(* Logix 5000 AddOnInstructionDefinition export Banner_Q90R2KU_Param_v4; software revision 33.00; part 2 of 3 *)
(* tags used below, declared in another part *)
   Q90RKU : Banner_Q90R2KU_v4;
   Port_Data : Banner_IOL_Port_v4;
   Port : DINT;
   Local_Control : DINT;
   Command_Being_Processed : BOOL;
   Update_Archive : BOOL;
   Index_Write_Inprocess : DINT;
   Index_Write_Control : DINT;
   Inprocess_Index : DINT;
(* Banner_Q90R2KU_Param_v4, continued *)

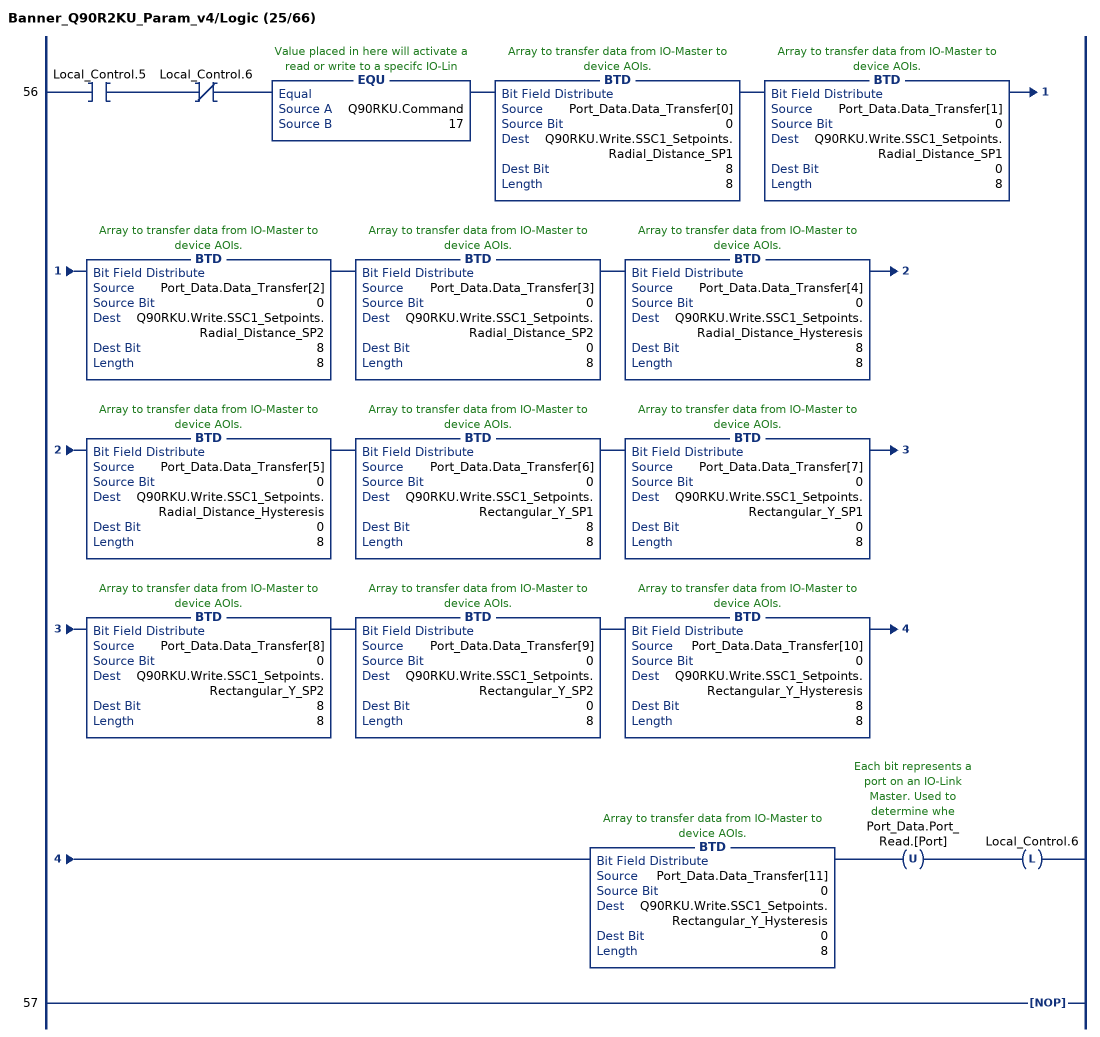
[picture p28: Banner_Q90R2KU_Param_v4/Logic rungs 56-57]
   56: XIC(Local_Control.5)XIO(Local_Control.6)EQU(Q90RKU.Command,17)BTD(Port_Data.Data_Transfer[0],0,Q90RKU.Write.SSC1_Setpoints.Radial_Distance_SP1,8,8)BTD(Port_Data.Data_Transfer[1],0,Q90RKU.Write.SSC1_Setpoints.Radial_Distance_SP1,0,8)BTD(Port_Data.Data_Transfer[2],0,Q90RKU.Write.SSC1_Setpoints.Radial_Distance_SP2,8,8)BTD(Port_Data.Data_Transfer[3],0,Q90RKU.Write.SSC1_Setpoints.Radial_Distance_SP2,0,8)BTD(Port_Data.Data_Transfer[4],0,Q90RKU.Write.SSC1_Setpoints.Radial_Distance_Hysteresis,8,8)BTD(Port_Data.Data_Transfer[5],0,Q90RKU.Write.SSC1_Setpoints.Radial_Distance_Hysteresis,0,8)BTD(Port_Data.Data_Transfer[6],0,Q90RKU.Write.SSC1_Setpoints.Rectangular_Y_SP1,8,8)BTD(Port_Data.Data_Transfer[7],0,Q90RKU.Write.SSC1_Setpoints.Rectangular_Y_SP1,0,8)BTD(Port_Data.Data_Transfer[8],0,Q90RKU.Write.SSC1_Setpoints.Rectangular_Y_SP2,8,8)BTD(Port_Data.Data_Transfer[9],0,Q90RKU.Write.SSC1_Setpoints.Rectangular_Y_SP2,0,8)BTD(Port_Data.Data_Transfer[10],0,Q90RKU.Write.SSC1_Setpoints.Rectangular_Y_Hysteresis,8,8)BTD(Port_Data.Data_Transfer[11],0,Q90RKU.Write.SSC1_Setpoints.Rectangular_Y_Hysteresis,0,8)OTU(Port_Data.Port_Read.[Port])OTL(Local_Control.6);
   57: NOP();
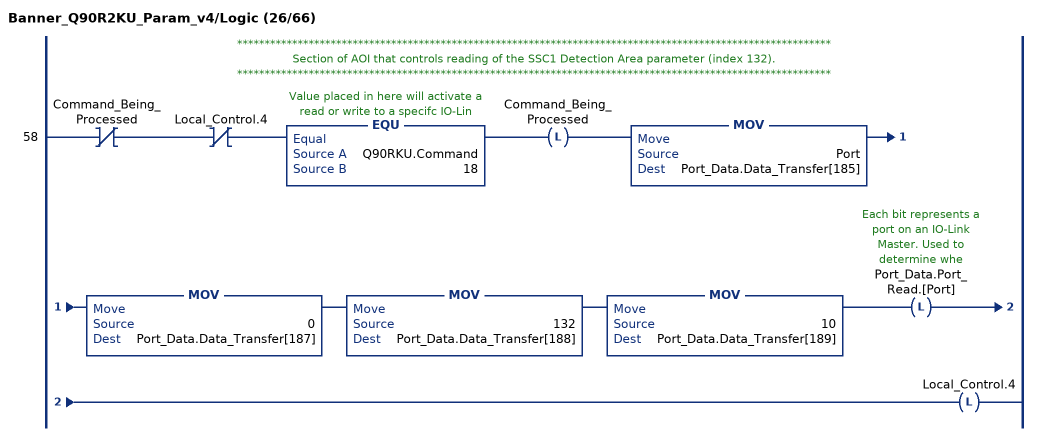
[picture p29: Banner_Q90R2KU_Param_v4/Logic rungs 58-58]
   // ************************************************************************************************************
   // Section of AOI that controls reading of the SSC1 Detection Area parameter (index 132).
   // ************************************************************************************************************
   58: XIO(Command_Being_Processed)XIO(Local_Control.4)EQU(Q90RKU.Command,18)OTL(Command_Being_Processed)MOV(Port,Port_Data.Data_Transfer[185])MOV(0,Port_Data.Data_Transfer[187])MOV(132,Port_Data.Data_Transfer[188])MOV(10,Port_Data.Data_Transfer[189])OTL(Port_Data.Port_Read.[Port])OTL(Local_Control.4);
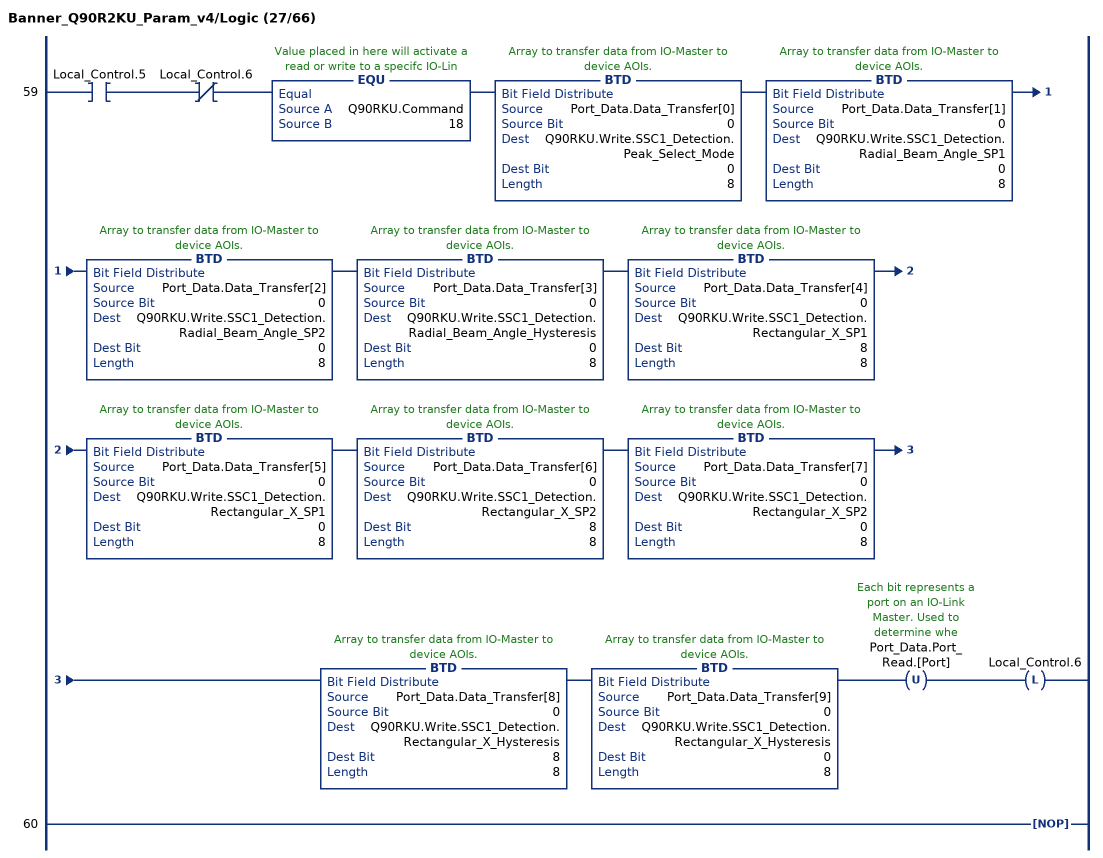
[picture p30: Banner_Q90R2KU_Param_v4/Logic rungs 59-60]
   59: XIC(Local_Control.5)XIO(Local_Control.6)EQU(Q90RKU.Command,18)BTD(Port_Data.Data_Transfer[0],0,Q90RKU.Write.SSC1_Detection.Peak_Select_Mode,0,8)BTD(Port_Data.Data_Transfer[1],0,Q90RKU.Write.SSC1_Detection.Radial_Beam_Angle_SP1,0,8)BTD(Port_Data.Data_Transfer[2],0,Q90RKU.Write.SSC1_Detection.Radial_Beam_Angle_SP2,0,8)BTD(Port_Data.Data_Transfer[3],0,Q90RKU.Write.SSC1_Detection.Radial_Beam_Angle_Hysteresis,0,8)BTD(Port_Data.Data_Transfer[4],0,Q90RKU.Write.SSC1_Detection.Rectangular_X_SP1,8,8)BTD(Port_Data.Data_Transfer[5],0,Q90RKU.Write.SSC1_Detection.Rectangular_X_SP1,0,8)BTD(Port_Data.Data_Transfer[6],0,Q90RKU.Write.SSC1_Detection.Rectangular_X_SP2,8,8)BTD(Port_Data.Data_Transfer[7],0,Q90RKU.Write.SSC1_Detection.Rectangular_X_SP2,0,8)BTD(Port_Data.Data_Transfer[8],0,Q90RKU.Write.SSC1_Detection.Rectangular_X_Hysteresis,8,8)BTD(Port_Data.Data_Transfer[9],0,Q90RKU.Write.SSC1_Detection.Rectangular_X_Hysteresis,0,8)OTU(Port_Data.Port_Read.[Port])OTL(Local_Control.6);
   60: NOP();
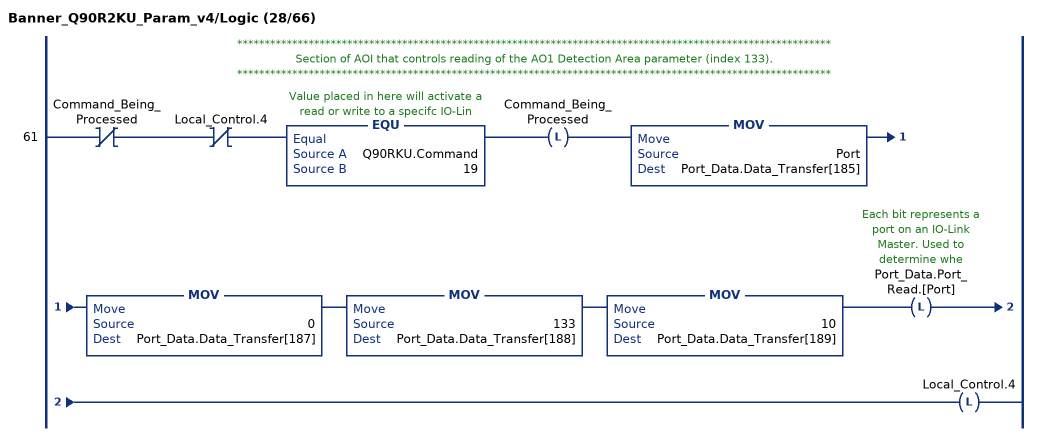
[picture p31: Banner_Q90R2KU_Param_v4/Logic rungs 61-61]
   // ************************************************************************************************************
   // Section of AOI that controls reading of the AO1 Detection Area parameter (index 133).
   // ************************************************************************************************************
   61: XIO(Command_Being_Processed)XIO(Local_Control.4)EQU(Q90RKU.Command,19)OTL(Command_Being_Processed)MOV(Port,Port_Data.Data_Transfer[185])MOV(0,Port_Data.Data_Transfer[187])MOV(133,Port_Data.Data_Transfer[188])MOV(10,Port_Data.Data_Transfer[189])OTL(Port_Data.Port_Read.[Port])OTL(Local_Control.4);
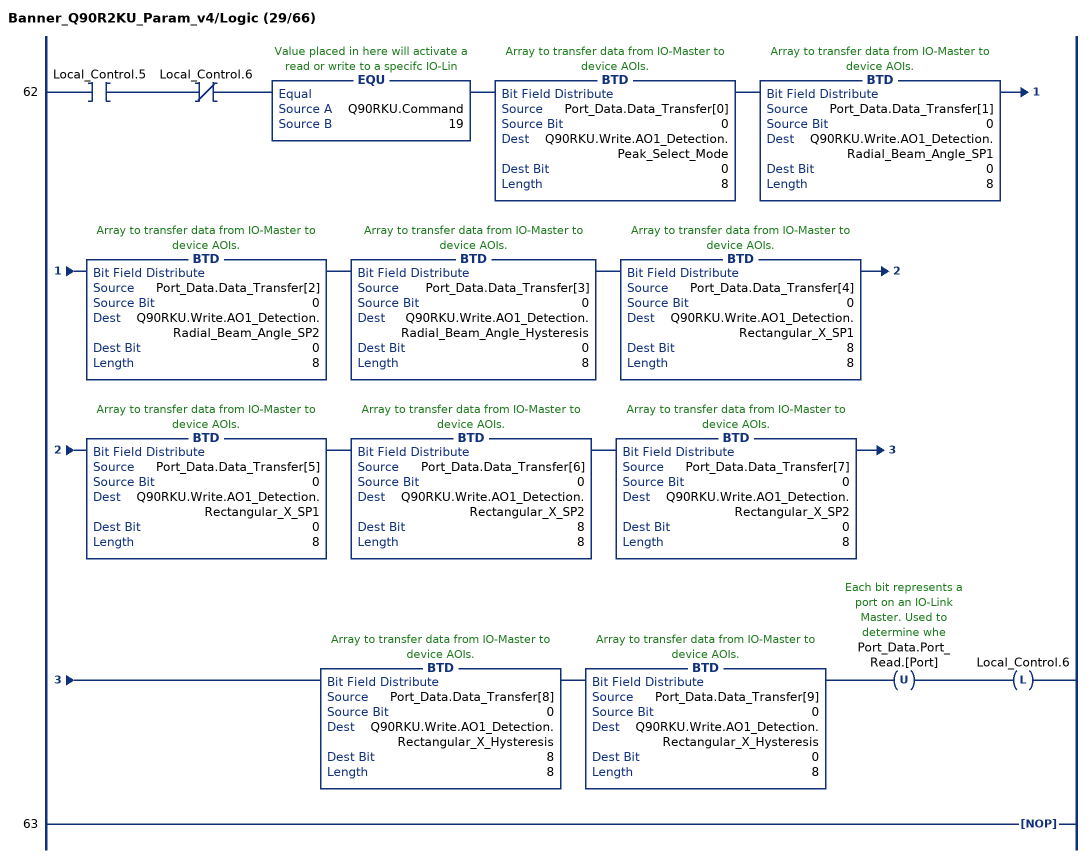
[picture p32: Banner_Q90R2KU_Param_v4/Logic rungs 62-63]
   62: XIC(Local_Control.5)XIO(Local_Control.6)EQU(Q90RKU.Command,19)BTD(Port_Data.Data_Transfer[0],0,Q90RKU.Write.AO1_Detection.Peak_Select_Mode,0,8)BTD(Port_Data.Data_Transfer[1],0,Q90RKU.Write.AO1_Detection.Radial_Beam_Angle_SP1,0,8)BTD(Port_Data.Data_Transfer[2],0,Q90RKU.Write.AO1_Detection.Radial_Beam_Angle_SP2,0,8)BTD(Port_Data.Data_Transfer[3],0,Q90RKU.Write.AO1_Detection.Radial_Beam_Angle_Hysteresis,0,8)BTD(Port_Data.Data_Transfer[4],0,Q90RKU.Write.AO1_Detection.Rectangular_X_SP1,8,8)BTD(Port_Data.Data_Transfer[5],0,Q90RKU.Write.AO1_Detection.Rectangular_X_SP1,0,8)BTD(Port_Data.Data_Transfer[6],0,Q90RKU.Write.AO1_Detection.Rectangular_X_SP2,8,8)BTD(Port_Data.Data_Transfer[7],0,Q90RKU.Write.AO1_Detection.Rectangular_X_SP2,0,8)BTD(Port_Data.Data_Transfer[8],0,Q90RKU.Write.AO1_Detection.Rectangular_X_Hysteresis,8,8)BTD(Port_Data.Data_Transfer[9],0,Q90RKU.Write.AO1_Detection.Rectangular_X_Hysteresis,0,8)OTU(Port_Data.Port_Read.[Port])OTL(Local_Control.6);
   63: NOP();
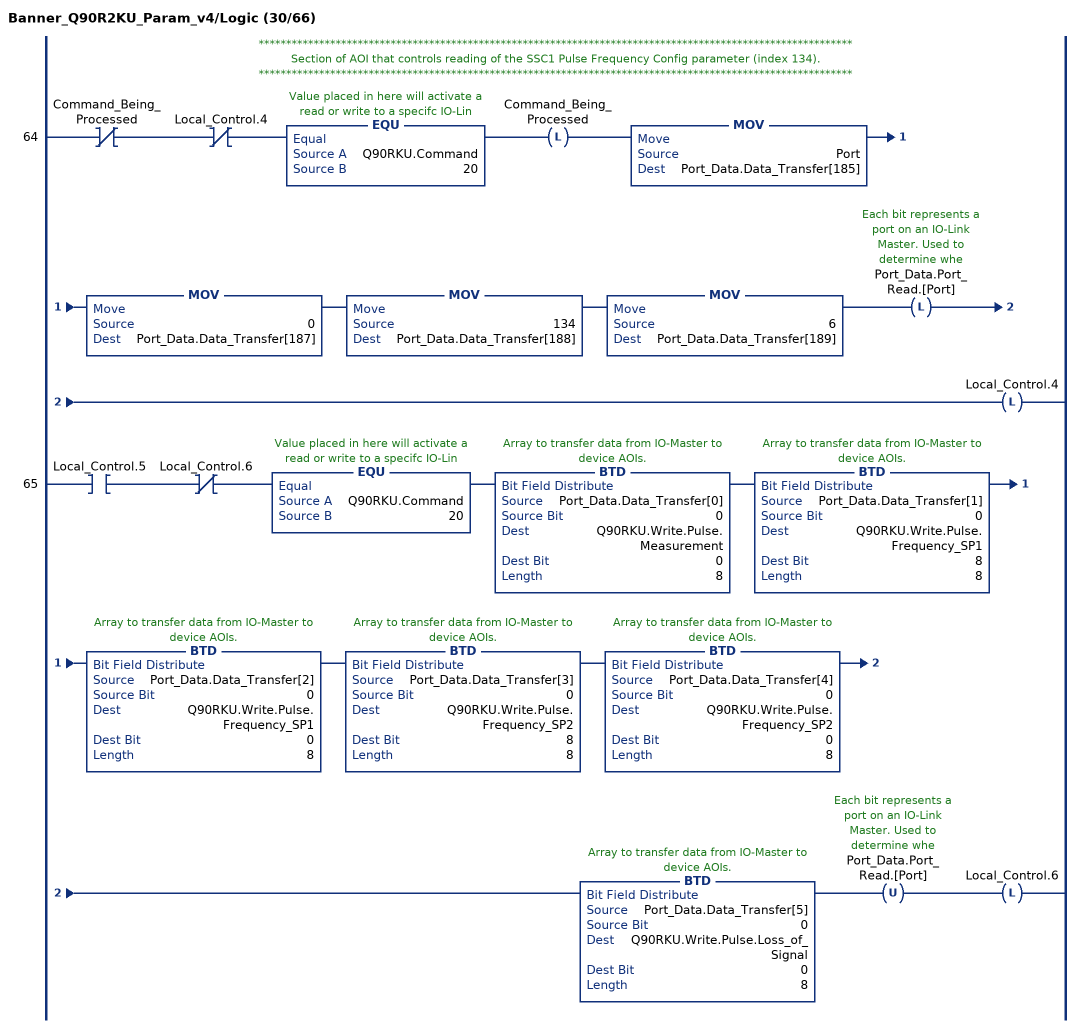
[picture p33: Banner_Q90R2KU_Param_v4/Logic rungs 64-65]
   // ************************************************************************************************************
   // Section of AOI that controls reading of the SSC1 Pulse Frequency Config parameter (index 134).
   // ************************************************************************************************************
   64: XIO(Command_Being_Processed)XIO(Local_Control.4)EQU(Q90RKU.Command,20)OTL(Command_Being_Processed)MOV(Port,Port_Data.Data_Transfer[185])MOV(0,Port_Data.Data_Transfer[187])MOV(134,Port_Data.Data_Transfer[188])MOV(6,Port_Data.Data_Transfer[189])OTL(Port_Data.Port_Read.[Port])OTL(Local_Control.4);
   65: XIC(Local_Control.5)XIO(Local_Control.6)EQU(Q90RKU.Command,20)BTD(Port_Data.Data_Transfer[0],0,Q90RKU.Write.Pulse.Measurement,0,8)BTD(Port_Data.Data_Transfer[1],0,Q90RKU.Write.Pulse.Frequency_SP1,8,8)BTD(Port_Data.Data_Transfer[2],0,Q90RKU.Write.Pulse.Frequency_SP1,0,8)BTD(Port_Data.Data_Transfer[3],0,Q90RKU.Write.Pulse.Frequency_SP2,8,8)BTD(Port_Data.Data_Transfer[4],0,Q90RKU.Write.Pulse.Frequency_SP2,0,8)BTD(Port_Data.Data_Transfer[5],0,Q90RKU.Write.Pulse.Loss_of_Signal,0,8)OTU(Port_Data.Port_Read.[Port])OTL(Local_Control.6);
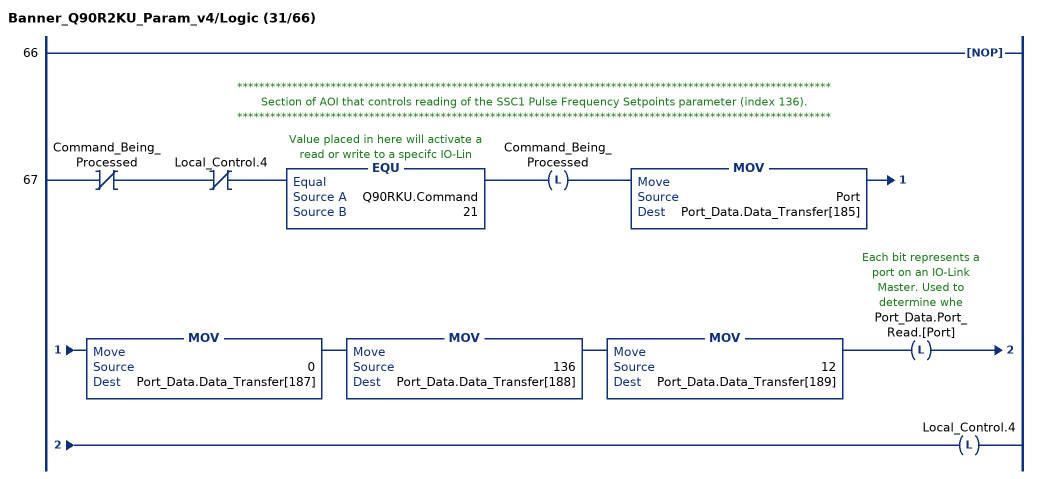
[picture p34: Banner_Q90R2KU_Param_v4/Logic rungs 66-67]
   66: NOP();
   // ************************************************************************************************************
   // Section of AOI that controls reading of the SSC1 Pulse Frequency Setpoints parameter (index 136).
   // ************************************************************************************************************
   67: XIO(Command_Being_Processed)XIO(Local_Control.4)EQU(Q90RKU.Command,21)OTL(Command_Being_Processed)MOV(Port,Port_Data.Data_Transfer[185])MOV(0,Port_Data.Data_Transfer[187])MOV(136,Port_Data.Data_Transfer[188])MOV(12,Port_Data.Data_Transfer[189])OTL(Port_Data.Port_Read.[Port])OTL(Local_Control.4);
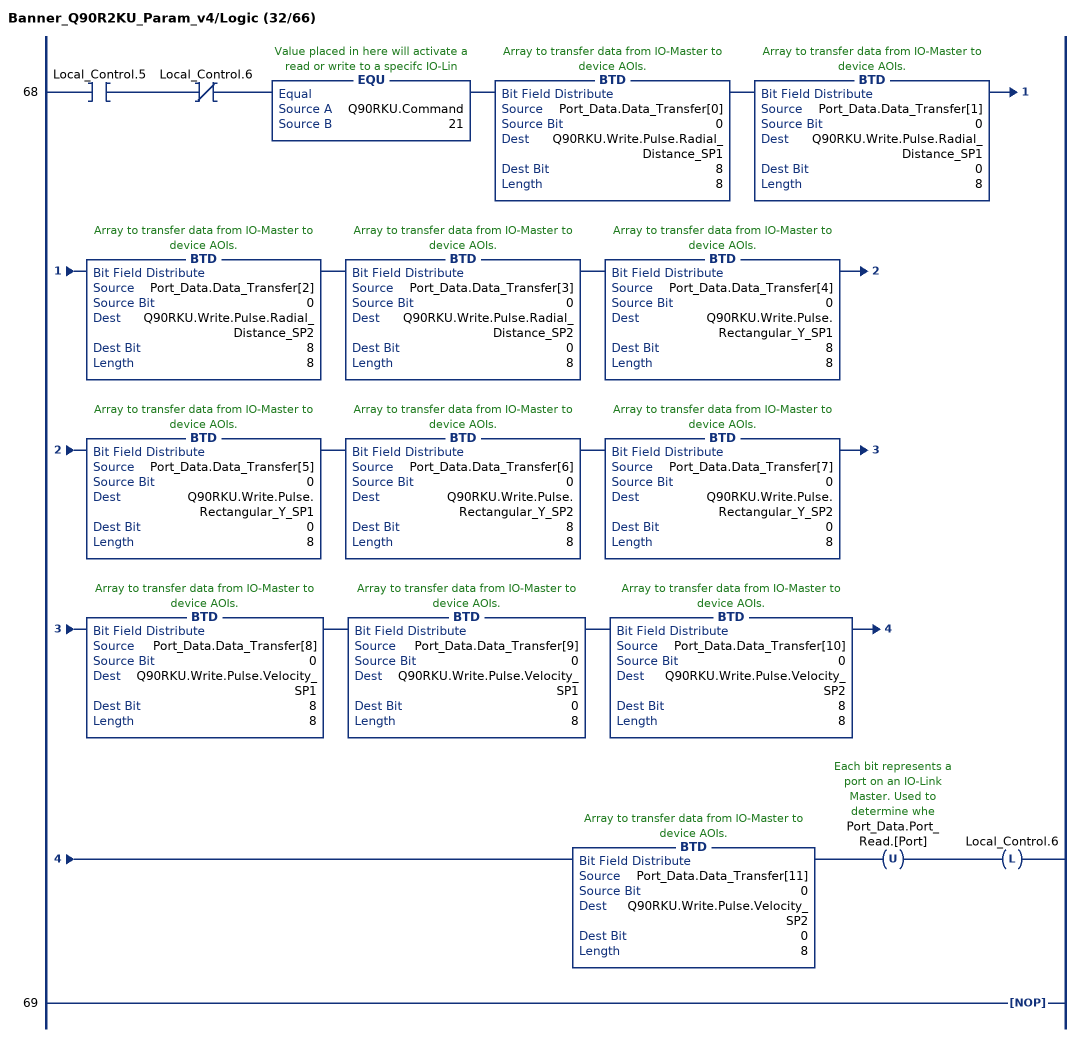
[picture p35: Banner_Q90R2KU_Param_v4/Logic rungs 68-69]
   68: XIC(Local_Control.5)XIO(Local_Control.6)EQU(Q90RKU.Command,21)BTD(Port_Data.Data_Transfer[0],0,Q90RKU.Write.Pulse.Radial_Distance_SP1,8,8)BTD(Port_Data.Data_Transfer[1],0,Q90RKU.Write.Pulse.Radial_Distance_SP1,0,8)BTD(Port_Data.Data_Transfer[2],0,Q90RKU.Write.Pulse.Radial_Distance_SP2,8,8)BTD(Port_Data.Data_Transfer[3],0,Q90RKU.Write.Pulse.Radial_Distance_SP2,0,8)BTD(Port_Data.Data_Transfer[4],0,Q90RKU.Write.Pulse.Rectangular_Y_SP1,8,8)BTD(Port_Data.Data_Transfer[5],0,Q90RKU.Write.Pulse.Rectangular_Y_SP1,0,8)BTD(Port_Data.Data_Transfer[6],0,Q90RKU.Write.Pulse.Rectangular_Y_SP2,8,8)BTD(Port_Data.Data_Transfer[7],0,Q90RKU.Write.Pulse.Rectangular_Y_SP2,0,8)BTD(Port_Data.Data_Transfer[8],0,Q90RKU.Write.Pulse.Velocity_SP1,8,8)BTD(Port_Data.Data_Transfer[9],0,Q90RKU.Write.Pulse.Velocity_SP1,0,8)BTD(Port_Data.Data_Transfer[10],0,Q90RKU.Write.Pulse.Velocity_SP2,8,8)BTD(Port_Data.Data_Transfer[11],0,Q90RKU.Write.Pulse.Velocity_SP2,0,8)OTU(Port_Data.Port_Read.[Port])OTL(Local_Control.6);
   69: NOP();
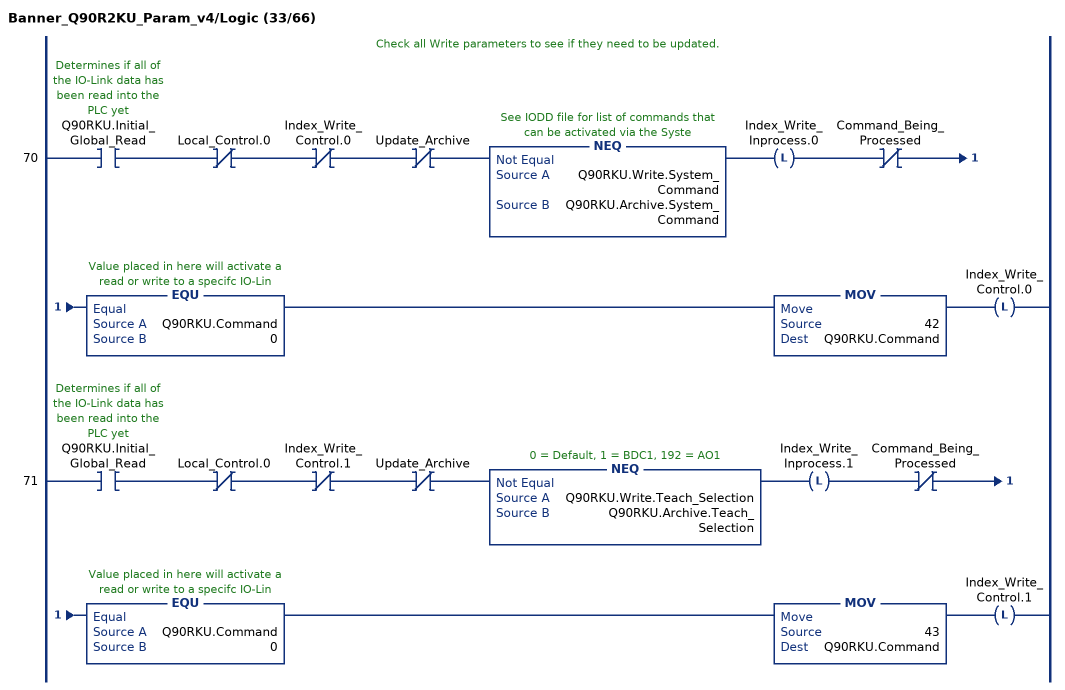
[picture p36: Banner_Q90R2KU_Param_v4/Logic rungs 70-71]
   // Check all Write parameters to see if they need to be updated.
   70: XIC(Q90RKU.Initial_Global_Read)XIO(Local_Control.0)XIO(Index_Write_Control.0)XIO(Update_Archive)NEQ(Q90RKU.Write.System_Command,Q90RKU.Archive.System_Command)OTL(Index_Write_Inprocess.0)XIO(Command_Being_Processed)EQU(Q90RKU.Command,0)MOV(42,Q90RKU.Command)OTL(Index_Write_Control.0);
   71: XIC(Q90RKU.Initial_Global_Read)XIO(Local_Control.0)XIO(Index_Write_Control.1)XIO(Update_Archive)NEQ(Q90RKU.Write.Teach_Selection,Q90RKU.Archive.Teach_Selection)OTL(Index_Write_Inprocess.1)XIO(Command_Being_Processed)EQU(Q90RKU.Command,0)MOV(43,Q90RKU.Command)OTL(Index_Write_Control.1);
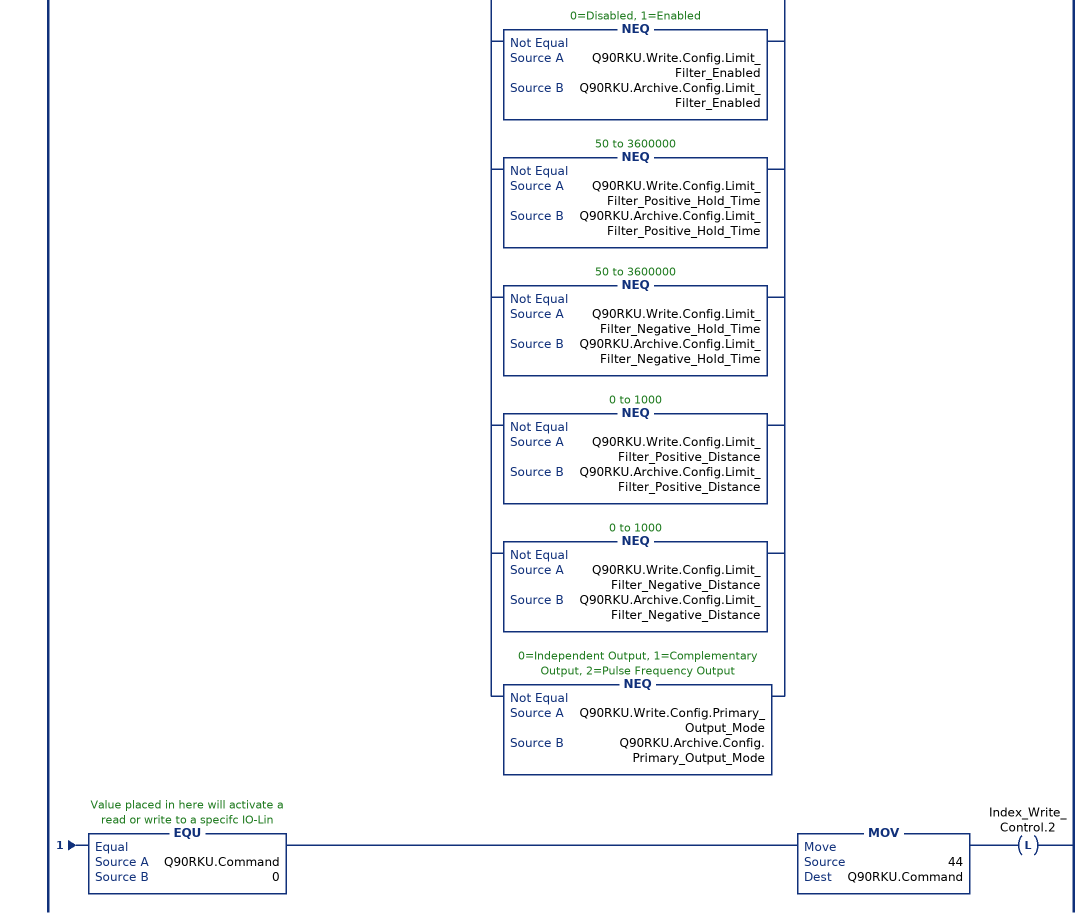
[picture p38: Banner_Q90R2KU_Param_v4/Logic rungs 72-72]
   72: XIC(Q90RKU.Initial_Global_Read)XIO(Local_Control.0)XIO(Index_Write_Control.2)XIO(Update_Archive)[NEQ(Q90RKU.Write.Config.Response_Speed,Q90RKU.Archive.Config.Response_Speed) ,NEQ(Q90RKU.Write.Config.Detection_Sensitivity,Q90RKU.Archive.Config.Detection_Sensitivity) ,NEQ(Q90RKU.Write.Config.LEDs_Disabled,Q90RKU.Archive.Config.LEDs_Disabled) ,NEQ(Q90RKU.Write.Config.Output_Polarity,Q90RKU.Archive.Config.Output_Polarity) ,NEQ(Q90RKU.Write.Config.PD_Measurement,Q90RKU.Archive.Config.PD_Measurement) ,NEQ(Q90RKU.Write.Config.Remote_Input_Mode,Q90RKU.Archive.Config.Remote_Input_Mode) ,NEQ(Q90RKU.Write.Config.Amplitude_Threshold,Q90RKU.Archive.Config.Amplitude_Threshold) ,NEQ(Q90RKU.Write.Config.Limit_Filter_Enabled,Q90RKU.Archive.Config.Limit_Filter_Enabled) ,NEQ(Q90RKU.Write.Config.Limit_Filter_Positive_Hold_Time,Q90RKU.Archive.Config.Limit_Filter_Positive_Hold_Time) ,NEQ(Q90RKU.Write.Config.Limit_Filter_Negative_Hold_Time,Q90RKU.Archive.Config.Limit_Filter_Negative_Hold_Time) ,NEQ(Q90RKU.Write.Config.Limit_Filter_Positive_Distance,Q90RKU.Archive.Config.Limit_Filter_Positive_Distance) ,NEQ(Q90RKU.Write.Config.Limit_Filter_Negative_Distance,Q90RKU.Archive.Config.Limit_Filter_Negative_Distance) ,NEQ(Q90RKU.Write.Config.Primary_Output_Mode,Q90RKU.Archive.Config.Primary_Output_Mode) ]OTL(Index_Write_Inprocess.2)XIO(Command_Being_Processed)EQU(Q90RKU.Command,0)MOV(44,Q90RKU.Command)OTL(Index_Write_Control.2);
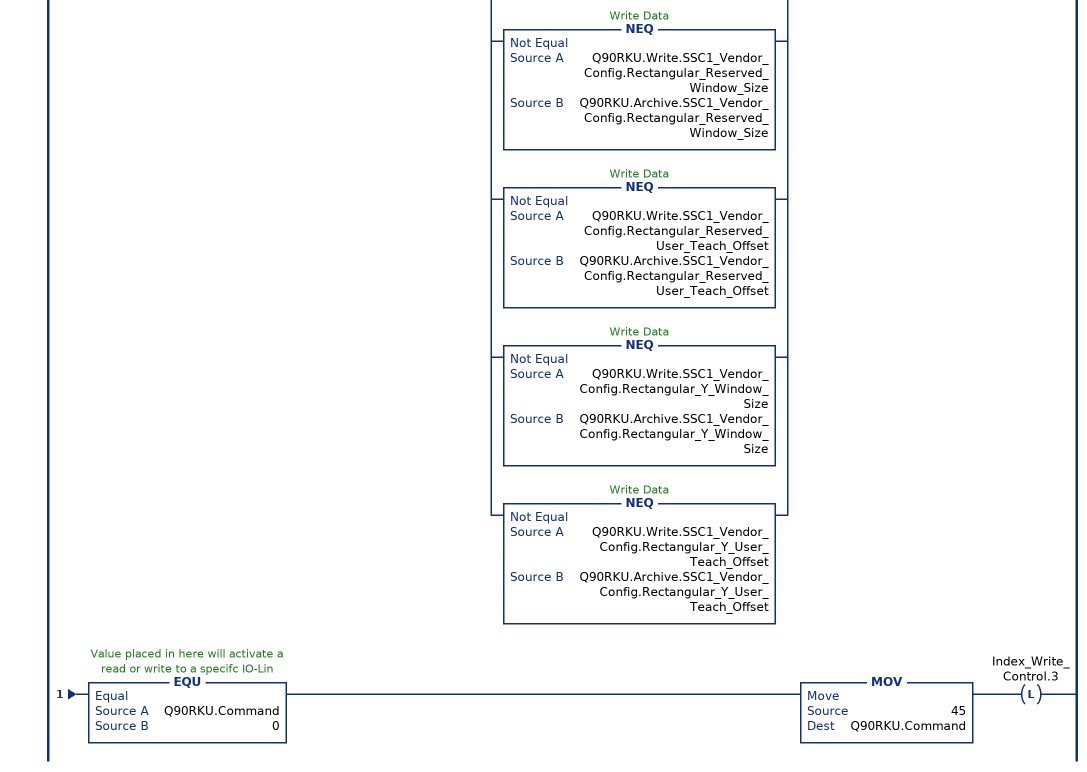
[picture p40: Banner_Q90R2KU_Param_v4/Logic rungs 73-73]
   73: XIC(Q90RKU.Initial_Global_Read)XIO(Local_Control.0)XIO(Index_Write_Control.3)XIO(Update_Archive)[NEQ(Q90RKU.Write.SSC1_Vendor_Config.Delay_On,Q90RKU.Archive.SSC1_Vendor_Config.Delay_On) ,NEQ(Q90RKU.Write.SSC1_Vendor_Config.Delay_Off,Q90RKU.Archive.SSC1_Vendor_Config.Delay_Off) ,NEQ(Q90RKU.Write.SSC1_Vendor_Config.Radial_Distance_Window_Size,Q90RKU.Archive.SSC1_Vendor_Config.Radial_Distance_Window_Size) ,NEQ(Q90RKU.Write.SSC1_Vendor_Config.Radial_Distance_User_Teach_Offset,Q90RKU.Archive.SSC1_Vendor_Config.Radial_Distance_User_Teach_Offset) ,NEQ(Q90RKU.Write.SSC1_Vendor_Config.Radial_Reserved_Window_Size,Q90RKU.Archive.SSC1_Vendor_Config.Radial_Reserved_Window_Size) ,NEQ(Q90RKU.Write.SSC1_Vendor_Config.Radial_Reserved_User_Teach_Offset,Q90RKU.Archive.SSC1_Vendor_Config.Radial_Reserved_User_Teach_Offset) ,NEQ(Q90RKU.Write.SSC1_Vendor_Config.Rectangular_Reserved_Window_Size,Q90RKU.Archive.SSC1_Vendor_Config.Rectangular_Reserved_Window_Size) ,NEQ(Q90RKU.Write.SSC1_Vendor_Config.Rectangular_Reserved_User_Teach_Offset,Q90RKU.Archive.SSC1_Vendor_Config.Rectangular_Reserved_User_Teach_Offset) ,NEQ(Q90RKU.Write.SSC1_Vendor_Config.Rectangular_Y_Window_Size,Q90RKU.Archive.SSC1_Vendor_Config.Rectangular_Y_Window_Size) ,NEQ(Q90RKU.Write.SSC1_Vendor_Config.Rectangular_Y_User_Teach_Offset,Q90RKU.Archive.SSC1_Vendor_Config.Rectangular_Y_User_Teach_Offset) ]OTL(Index_Write_Inprocess.3)XIO(Command_Being_Processed)EQU(Q90RKU.Command,0)MOV(45,Q90RKU.Command)OTL(Index_Write_Control.3);
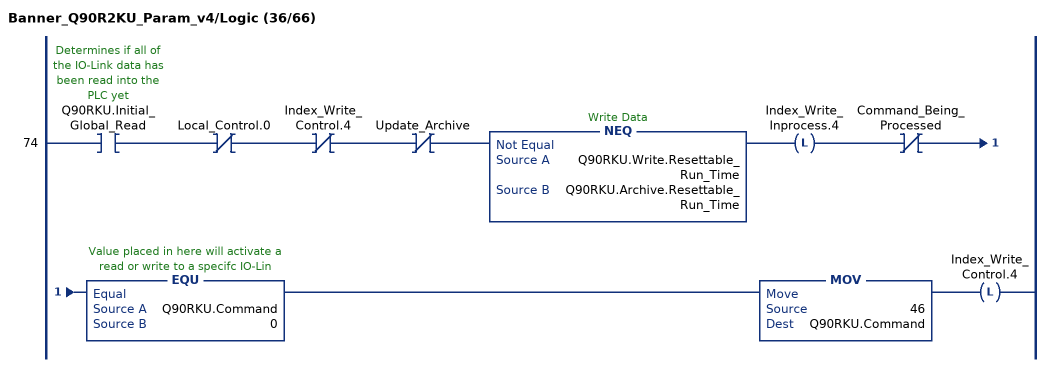
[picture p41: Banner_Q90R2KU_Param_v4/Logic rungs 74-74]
   74: XIC(Q90RKU.Initial_Global_Read)XIO(Local_Control.0)XIO(Index_Write_Control.4)XIO(Update_Archive)NEQ(Q90RKU.Write.Resettable_Run_Time,Q90RKU.Archive.Resettable_Run_Time)OTL(Index_Write_Inprocess.4)XIO(Command_Being_Processed)EQU(Q90RKU.Command,0)MOV(46,Q90RKU.Command)OTL(Index_Write_Control.4);
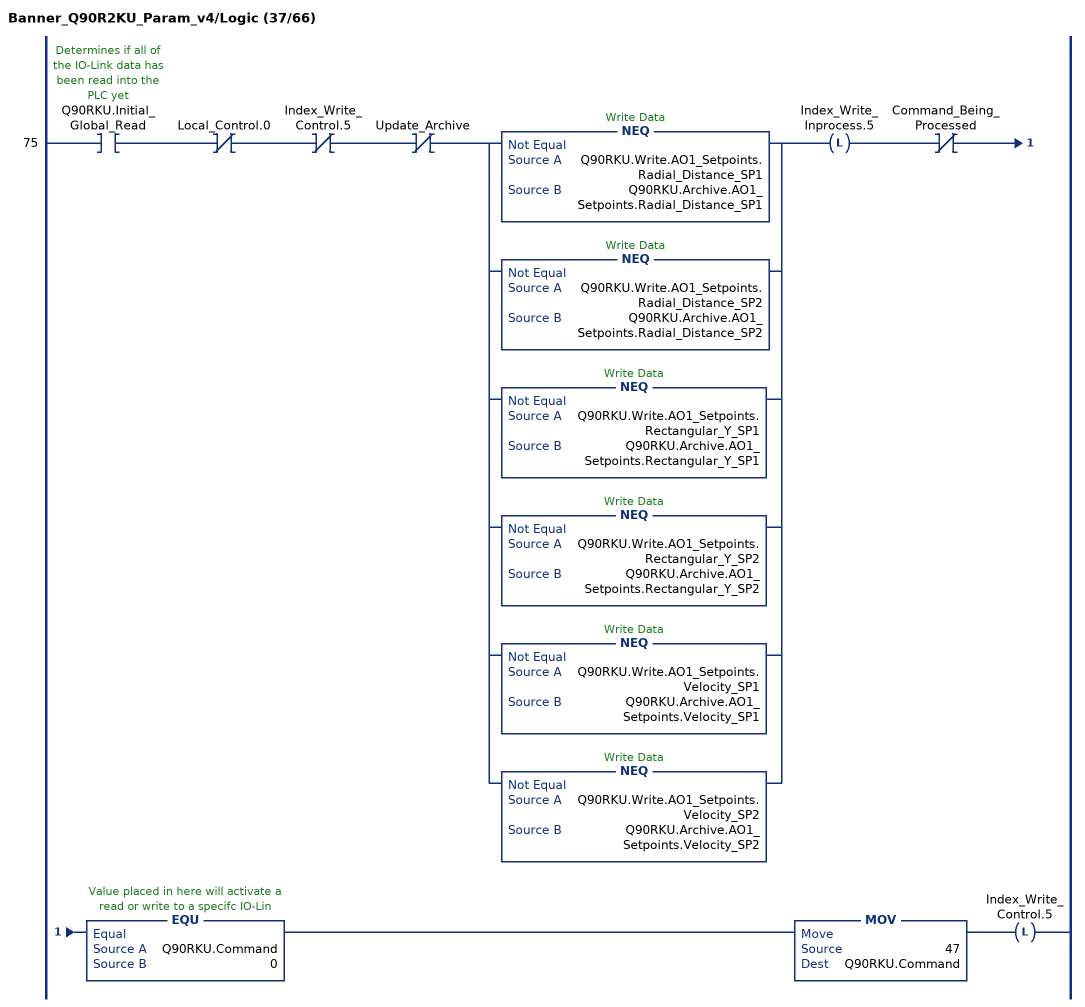
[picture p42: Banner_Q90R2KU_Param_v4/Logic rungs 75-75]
   75: XIC(Q90RKU.Initial_Global_Read)XIO(Local_Control.0)XIO(Index_Write_Control.5)XIO(Update_Archive)[NEQ(Q90RKU.Write.AO1_Setpoints.Radial_Distance_SP1,Q90RKU.Archive.AO1_Setpoints.Radial_Distance_SP1) ,NEQ(Q90RKU.Write.AO1_Setpoints.Radial_Distance_SP2,Q90RKU.Archive.AO1_Setpoints.Radial_Distance_SP2) ,NEQ(Q90RKU.Write.AO1_Setpoints.Rectangular_Y_SP1,Q90RKU.Archive.AO1_Setpoints.Rectangular_Y_SP1) ,NEQ(Q90RKU.Write.AO1_Setpoints.Rectangular_Y_SP2,Q90RKU.Archive.AO1_Setpoints.Rectangular_Y_SP2) ,NEQ(Q90RKU.Write.AO1_Setpoints.Velocity_SP1,Q90RKU.Archive.AO1_Setpoints.Velocity_SP1) ,NEQ(Q90RKU.Write.AO1_Setpoints.Velocity_SP2,Q90RKU.Archive.AO1_Setpoints.Velocity_SP2) ]OTL(Index_Write_Inprocess.5)XIO(Command_Being_Processed)EQU(Q90RKU.Command,0)MOV(47,Q90RKU.Command)OTL(Index_Write_Control.5);
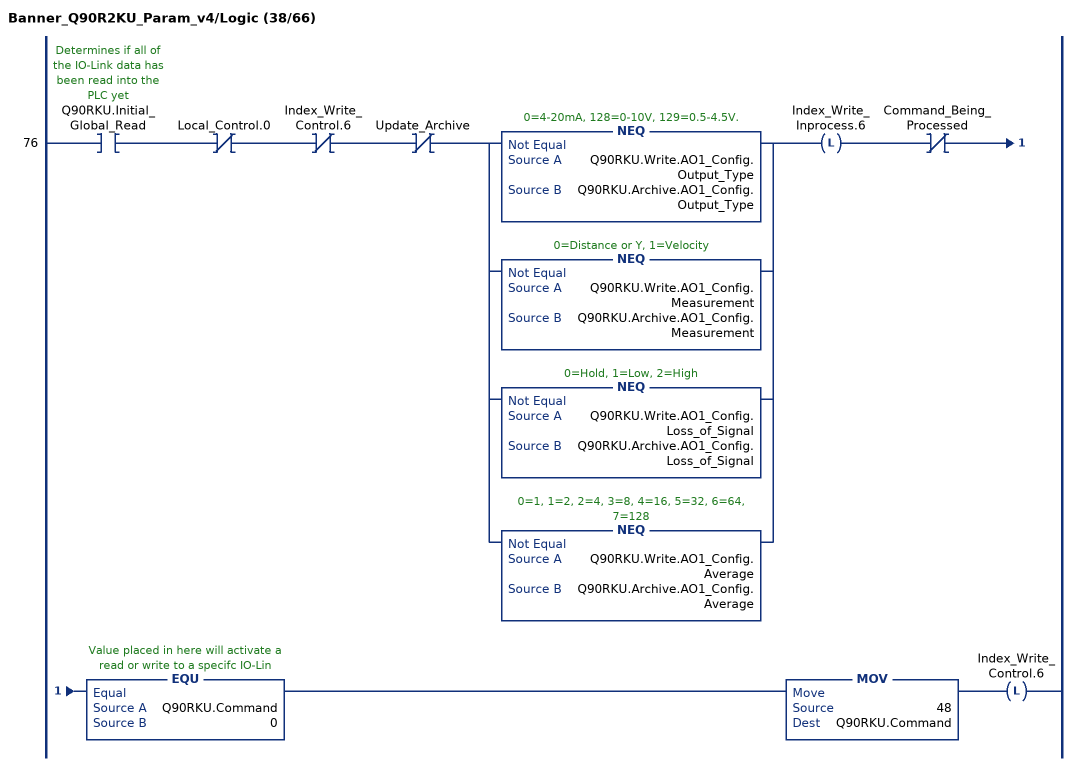
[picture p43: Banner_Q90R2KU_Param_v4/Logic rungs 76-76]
   76: XIC(Q90RKU.Initial_Global_Read)XIO(Local_Control.0)XIO(Index_Write_Control.6)XIO(Update_Archive)[NEQ(Q90RKU.Write.AO1_Config.Output_Type,Q90RKU.Archive.AO1_Config.Output_Type) ,NEQ(Q90RKU.Write.AO1_Config.Measurement,Q90RKU.Archive.AO1_Config.Measurement) ,NEQ(Q90RKU.Write.AO1_Config.Loss_of_Signal,Q90RKU.Archive.AO1_Config.Loss_of_Signal) ,NEQ(Q90RKU.Write.AO1_Config.Average,Q90RKU.Archive.AO1_Config.Average) ]OTL(Index_Write_Inprocess.6)XIO(Command_Being_Processed)EQU(Q90RKU.Command,0)MOV(48,Q90RKU.Command)OTL(Index_Write_Control.6);
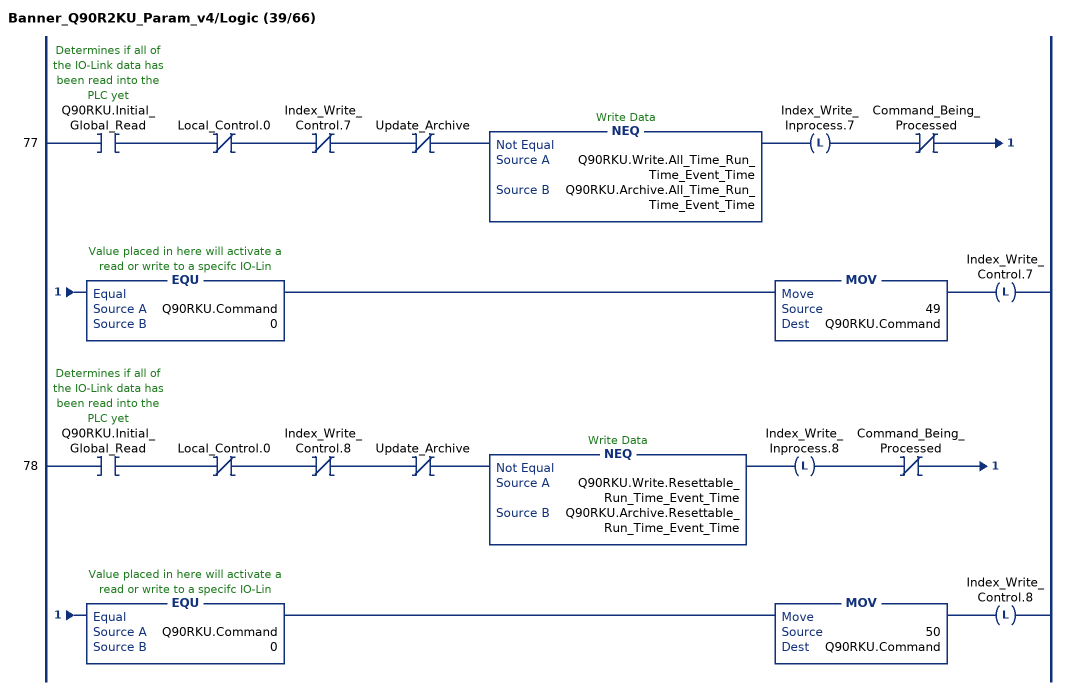
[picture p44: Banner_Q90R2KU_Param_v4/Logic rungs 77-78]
   77: XIC(Q90RKU.Initial_Global_Read)XIO(Local_Control.0)XIO(Index_Write_Control.7)XIO(Update_Archive)NEQ(Q90RKU.Write.All_Time_Run_Time_Event_Time,Q90RKU.Archive.All_Time_Run_Time_Event_Time)OTL(Index_Write_Inprocess.7)XIO(Command_Being_Processed)EQU(Q90RKU.Command,0)MOV(49,Q90RKU.Command)OTL(Index_Write_Control.7);
   78: XIC(Q90RKU.Initial_Global_Read)XIO(Local_Control.0)XIO(Index_Write_Control.8)XIO(Update_Archive)NEQ(Q90RKU.Write.Resettable_Run_Time_Event_Time,Q90RKU.Archive.Resettable_Run_Time_Event_Time)OTL(Index_Write_Inprocess.8)XIO(Command_Being_Processed)EQU(Q90RKU.Command,0)MOV(50,Q90RKU.Command)OTL(Index_Write_Control.8);
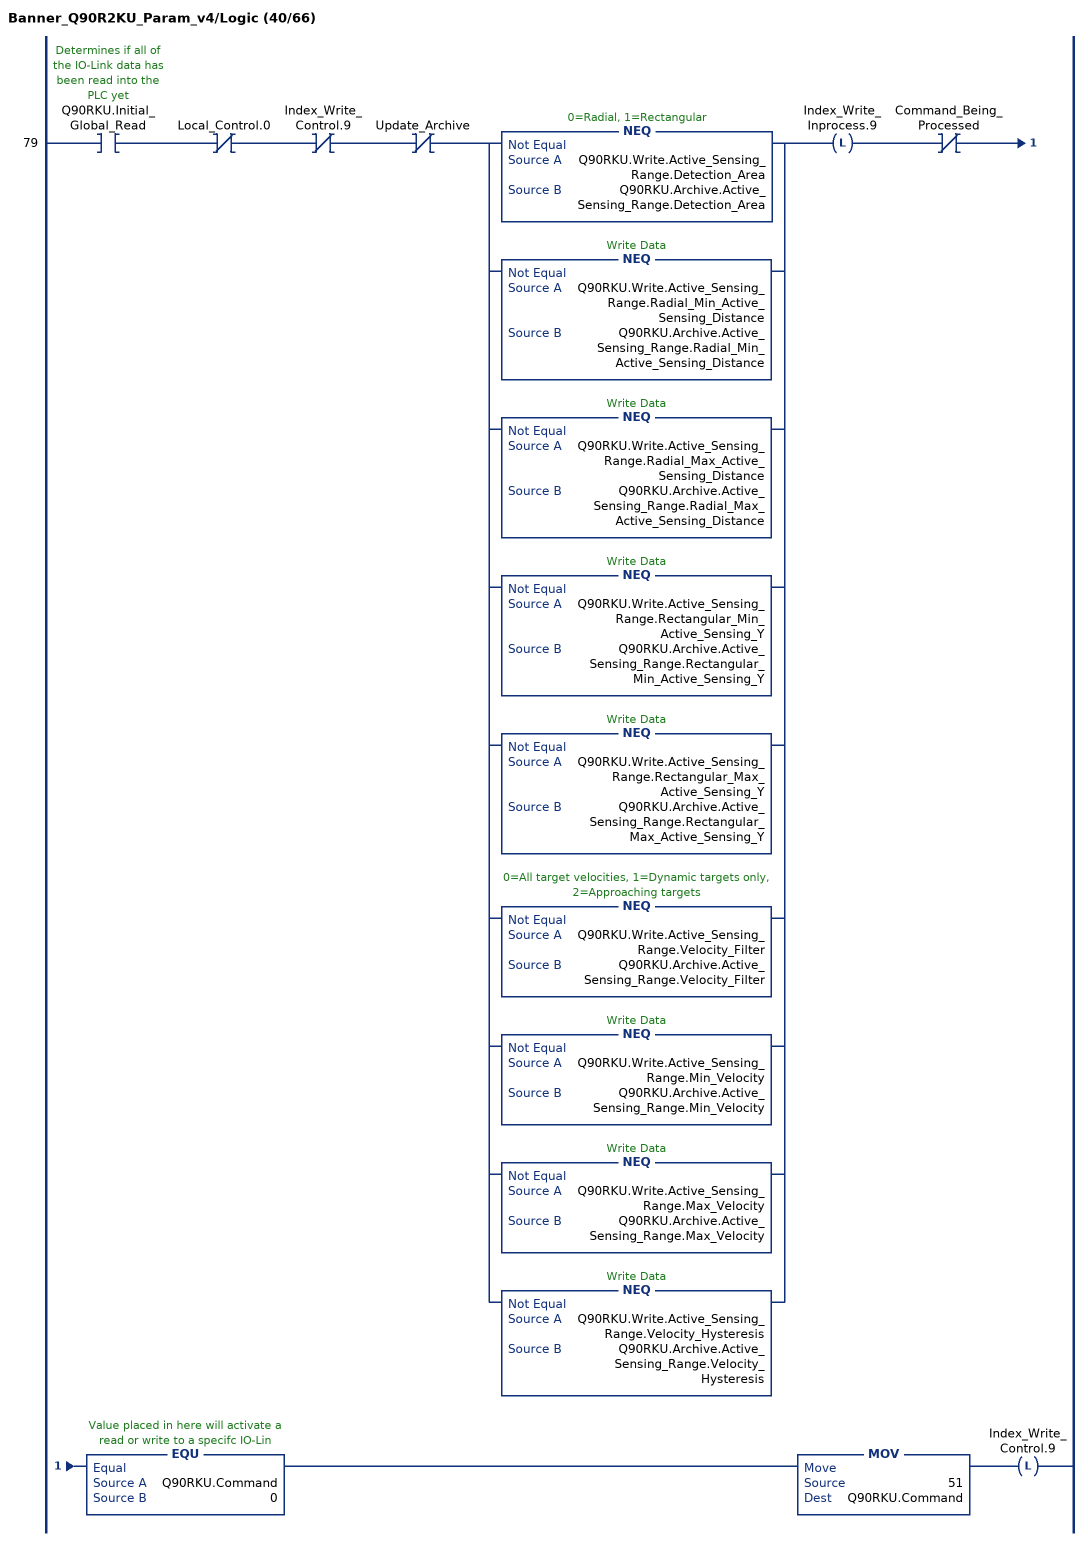
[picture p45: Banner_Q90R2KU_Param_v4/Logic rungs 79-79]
   79: XIC(Q90RKU.Initial_Global_Read)XIO(Local_Control.0)XIO(Index_Write_Control.9)XIO(Update_Archive)[NEQ(Q90RKU.Write.Active_Sensing_Range.Detection_Area,Q90RKU.Archive.Active_Sensing_Range.Detection_Area) ,NEQ(Q90RKU.Write.Active_Sensing_Range.Radial_Min_Active_Sensing_Distance,Q90RKU.Archive.Active_Sensing_Range.Radial_Min_Active_Sensing_Distance) ,NEQ(Q90RKU.Write.Active_Sensing_Range.Radial_Max_Active_Sensing_Distance,Q90RKU.Archive.Active_Sensing_Range.Radial_Max_Active_Sensing_Distance) ,NEQ(Q90RKU.Write.Active_Sensing_Range.Rectangular_Min_Active_Sensing_Y,Q90RKU.Archive.Active_Sensing_Range.Rectangular_Min_Active_Sensing_Y) ,NEQ(Q90RKU.Write.Active_Sensing_Range.Rectangular_Max_Active_Sensing_Y,Q90RKU.Archive.Active_Sensing_Range.Rectangular_Max_Active_Sensing_Y) ,NEQ(Q90RKU.Write.Active_Sensing_Range.Velocity_Filter,Q90RKU.Archive.Active_Sensing_Range.Velocity_Filter) ,NEQ(Q90RKU.Write.Active_Sensing_Range.Min_Velocity,Q90RKU.Archive.Active_Sensing_Range.Min_Velocity) ,NEQ(Q90RKU.Write.Active_Sensing_Range.Max_Velocity,Q90RKU.Archive.Active_Sensing_Range.Max_Velocity) ,NEQ(Q90RKU.Write.Active_Sensing_Range.Velocity_Hysteresis,Q90RKU.Archive.Active_Sensing_Range.Velocity_Hysteresis) ]OTL(Index_Write_Inprocess.9)XIO(Command_Being_Processed)EQU(Q90RKU.Command,0)MOV(51,Q90RKU.Command)OTL(Index_Write_Control.9);
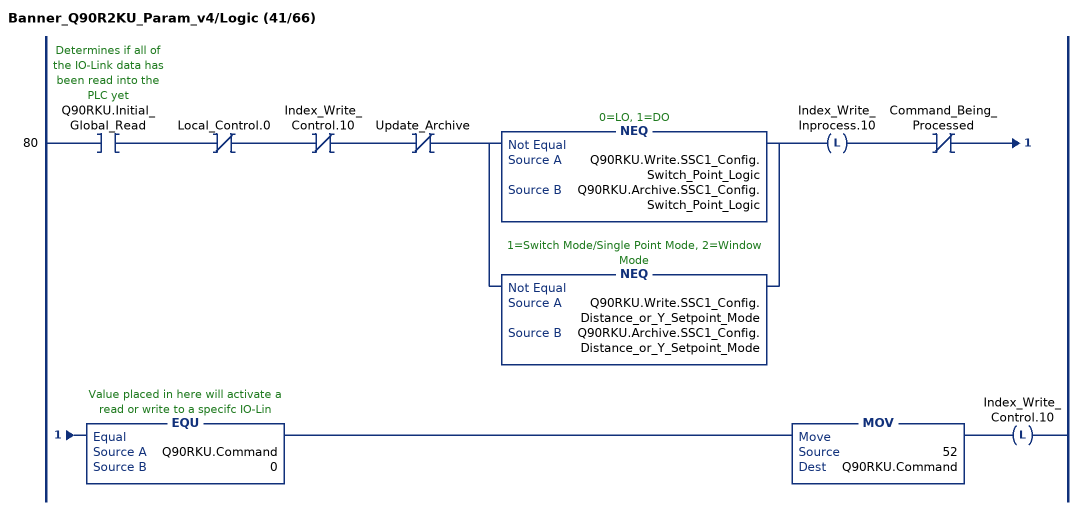
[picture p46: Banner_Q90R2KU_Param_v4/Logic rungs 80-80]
   80: XIC(Q90RKU.Initial_Global_Read)XIO(Local_Control.0)XIO(Index_Write_Control.10)XIO(Update_Archive)[NEQ(Q90RKU.Write.SSC1_Config.Switch_Point_Logic,Q90RKU.Archive.SSC1_Config.Switch_Point_Logic) ,NEQ(Q90RKU.Write.SSC1_Config.Distance_or_Y_Setpoint_Mode,Q90RKU.Archive.SSC1_Config.Distance_or_Y_Setpoint_Mode) ]OTL(Index_Write_Inprocess.10)XIO(Command_Being_Processed)EQU(Q90RKU.Command,0)MOV(52,Q90RKU.Command)OTL(Index_Write_Control.10);
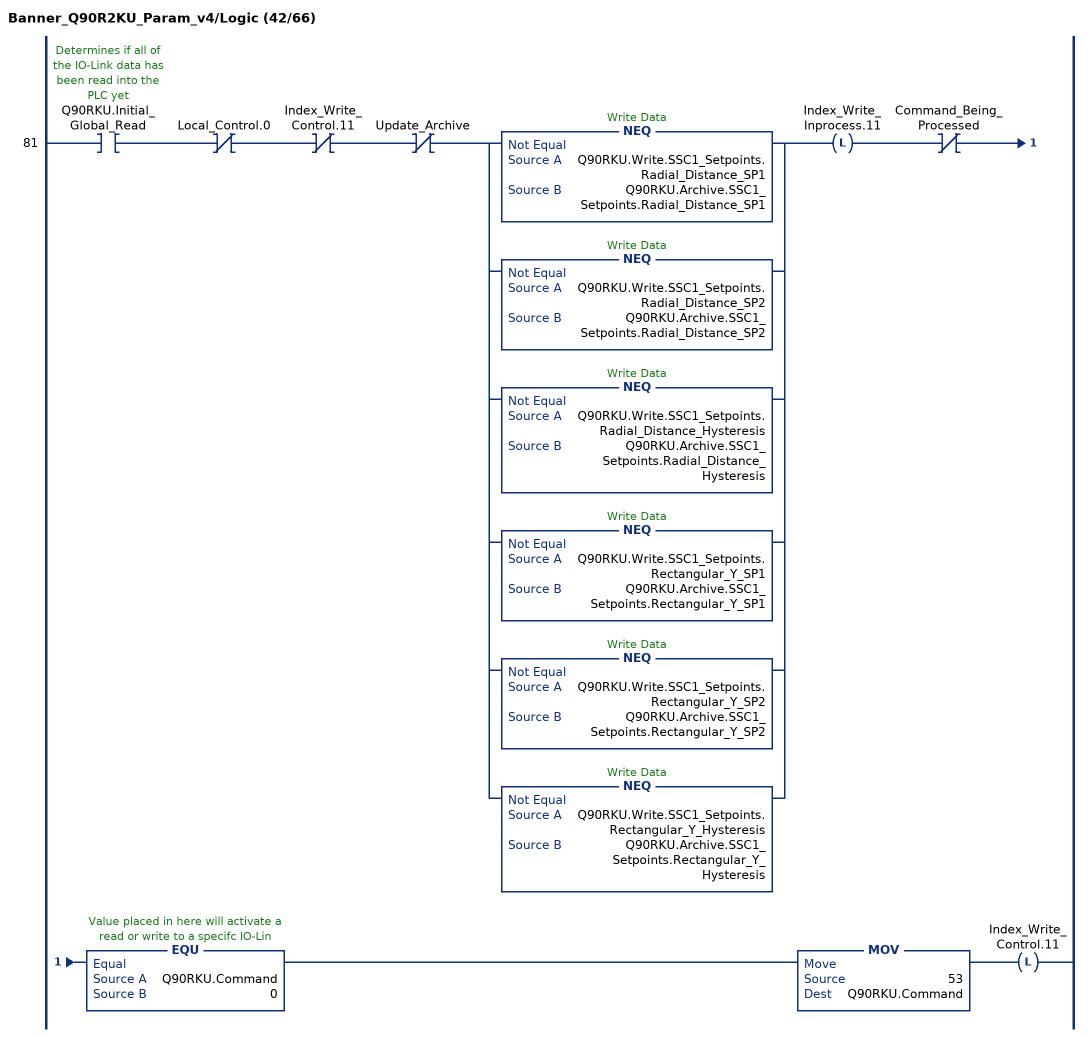
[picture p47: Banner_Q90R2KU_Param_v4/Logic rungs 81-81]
   81: XIC(Q90RKU.Initial_Global_Read)XIO(Local_Control.0)XIO(Index_Write_Control.11)XIO(Update_Archive)[NEQ(Q90RKU.Write.SSC1_Setpoints.Radial_Distance_SP1,Q90RKU.Archive.SSC1_Setpoints.Radial_Distance_SP1) ,NEQ(Q90RKU.Write.SSC1_Setpoints.Radial_Distance_SP2,Q90RKU.Archive.SSC1_Setpoints.Radial_Distance_SP2) ,NEQ(Q90RKU.Write.SSC1_Setpoints.Radial_Distance_Hysteresis,Q90RKU.Archive.SSC1_Setpoints.Radial_Distance_Hysteresis) ,NEQ(Q90RKU.Write.SSC1_Setpoints.Rectangular_Y_SP1,Q90RKU.Archive.SSC1_Setpoints.Rectangular_Y_SP1) ,NEQ(Q90RKU.Write.SSC1_Setpoints.Rectangular_Y_SP2,Q90RKU.Archive.SSC1_Setpoints.Rectangular_Y_SP2) ,NEQ(Q90RKU.Write.SSC1_Setpoints.Rectangular_Y_Hysteresis,Q90RKU.Archive.SSC1_Setpoints.Rectangular_Y_Hysteresis) ]OTL(Index_Write_Inprocess.11)XIO(Command_Being_Processed)EQU(Q90RKU.Command,0)MOV(53,Q90RKU.Command)OTL(Index_Write_Control.11);
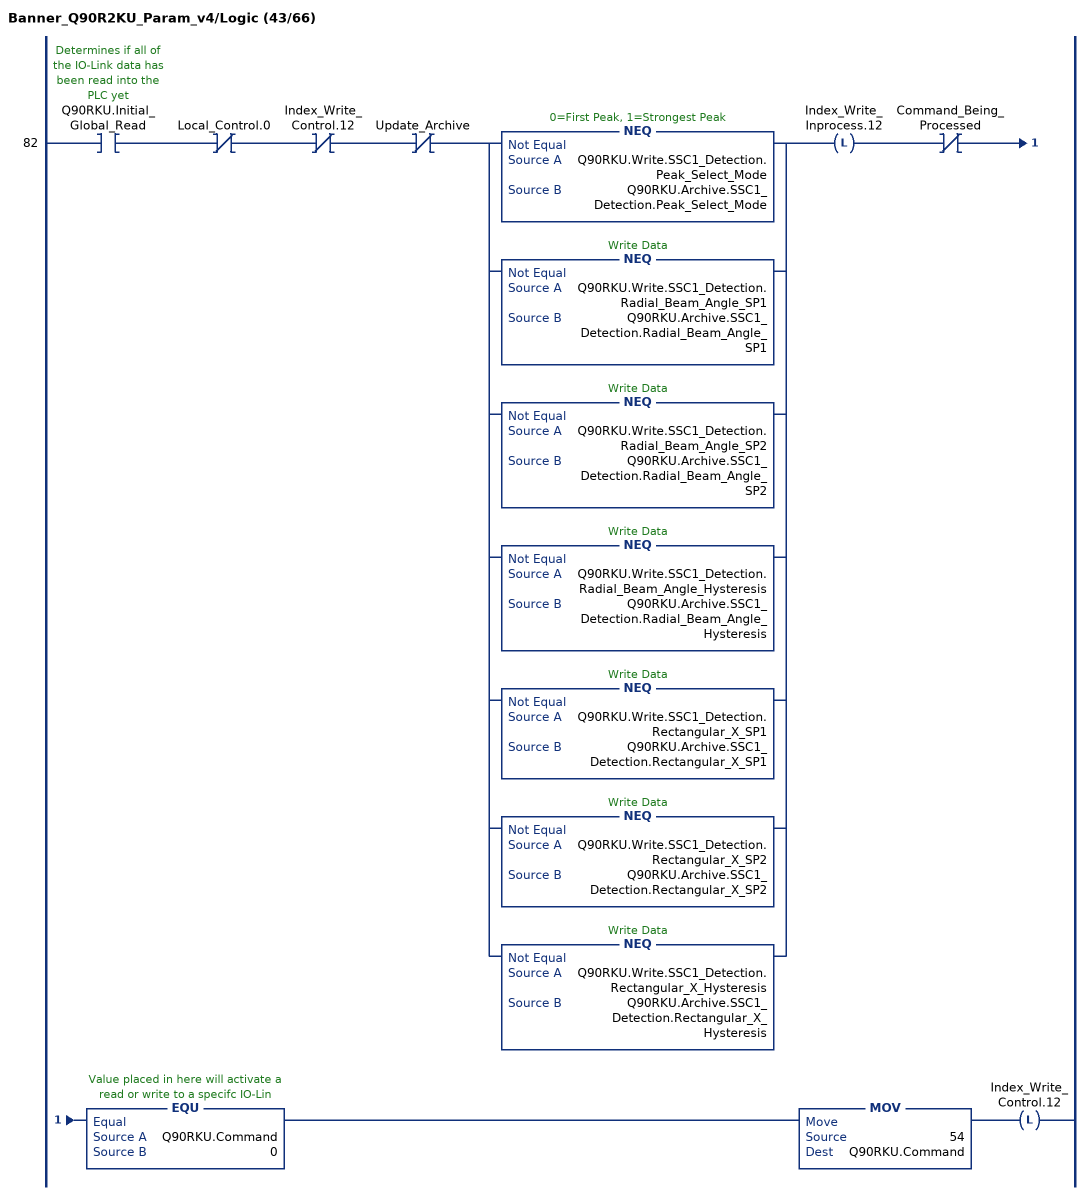
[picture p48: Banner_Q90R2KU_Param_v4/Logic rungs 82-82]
   82: XIC(Q90RKU.Initial_Global_Read)XIO(Local_Control.0)XIO(Index_Write_Control.12)XIO(Update_Archive)[NEQ(Q90RKU.Write.SSC1_Detection.Peak_Select_Mode,Q90RKU.Archive.SSC1_Detection.Peak_Select_Mode) ,NEQ(Q90RKU.Write.SSC1_Detection.Radial_Beam_Angle_SP1,Q90RKU.Archive.SSC1_Detection.Radial_Beam_Angle_SP1) ,NEQ(Q90RKU.Write.SSC1_Detection.Radial_Beam_Angle_SP2,Q90RKU.Archive.SSC1_Detection.Radial_Beam_Angle_SP2) ,NEQ(Q90RKU.Write.SSC1_Detection.Radial_Beam_Angle_Hysteresis,Q90RKU.Archive.SSC1_Detection.Radial_Beam_Angle_Hysteresis) ,NEQ(Q90RKU.Write.SSC1_Detection.Rectangular_X_SP1,Q90RKU.Archive.SSC1_Detection.Rectangular_X_SP1) ,NEQ(Q90RKU.Write.SSC1_Detection.Rectangular_X_SP2,Q90RKU.Archive.SSC1_Detection.Rectangular_X_SP2) ,NEQ(Q90RKU.Write.SSC1_Detection.Rectangular_X_Hysteresis,Q90RKU.Archive.SSC1_Detection.Rectangular_X_Hysteresis) ]OTL(Index_Write_Inprocess.12)XIO(Command_Being_Processed)EQU(Q90RKU.Command,0)MOV(54,Q90RKU.Command)OTL(Index_Write_Control.12);
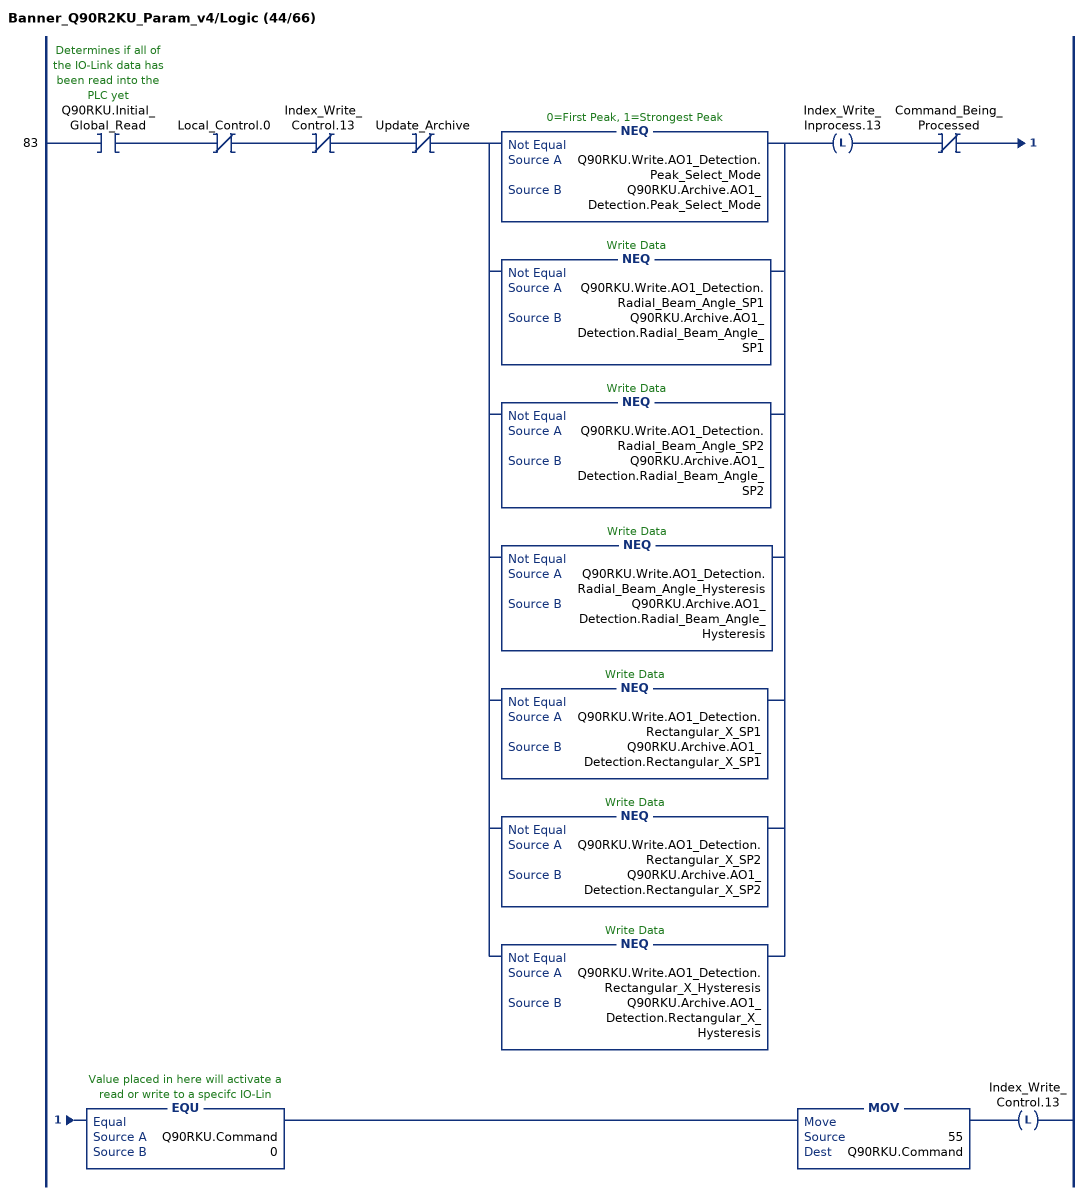
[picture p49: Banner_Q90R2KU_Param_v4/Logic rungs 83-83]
   83: XIC(Q90RKU.Initial_Global_Read)XIO(Local_Control.0)XIO(Index_Write_Control.13)XIO(Update_Archive)[NEQ(Q90RKU.Write.AO1_Detection.Peak_Select_Mode,Q90RKU.Archive.AO1_Detection.Peak_Select_Mode) ,NEQ(Q90RKU.Write.AO1_Detection.Radial_Beam_Angle_SP1,Q90RKU.Archive.AO1_Detection.Radial_Beam_Angle_SP1) ,NEQ(Q90RKU.Write.AO1_Detection.Radial_Beam_Angle_SP2,Q90RKU.Archive.AO1_Detection.Radial_Beam_Angle_SP2) ,NEQ(Q90RKU.Write.AO1_Detection.Radial_Beam_Angle_Hysteresis,Q90RKU.Archive.AO1_Detection.Radial_Beam_Angle_Hysteresis) ,NEQ(Q90RKU.Write.AO1_Detection.Rectangular_X_SP1,Q90RKU.Archive.AO1_Detection.Rectangular_X_SP1) ,NEQ(Q90RKU.Write.AO1_Detection.Rectangular_X_SP2,Q90RKU.Archive.AO1_Detection.Rectangular_X_SP2) ,NEQ(Q90RKU.Write.AO1_Detection.Rectangular_X_Hysteresis,Q90RKU.Archive.AO1_Detection.Rectangular_X_Hysteresis) ]OTL(Index_Write_Inprocess.13)XIO(Command_Being_Processed)EQU(Q90RKU.Command,0)MOV(55,Q90RKU.Command)OTL(Index_Write_Control.13);
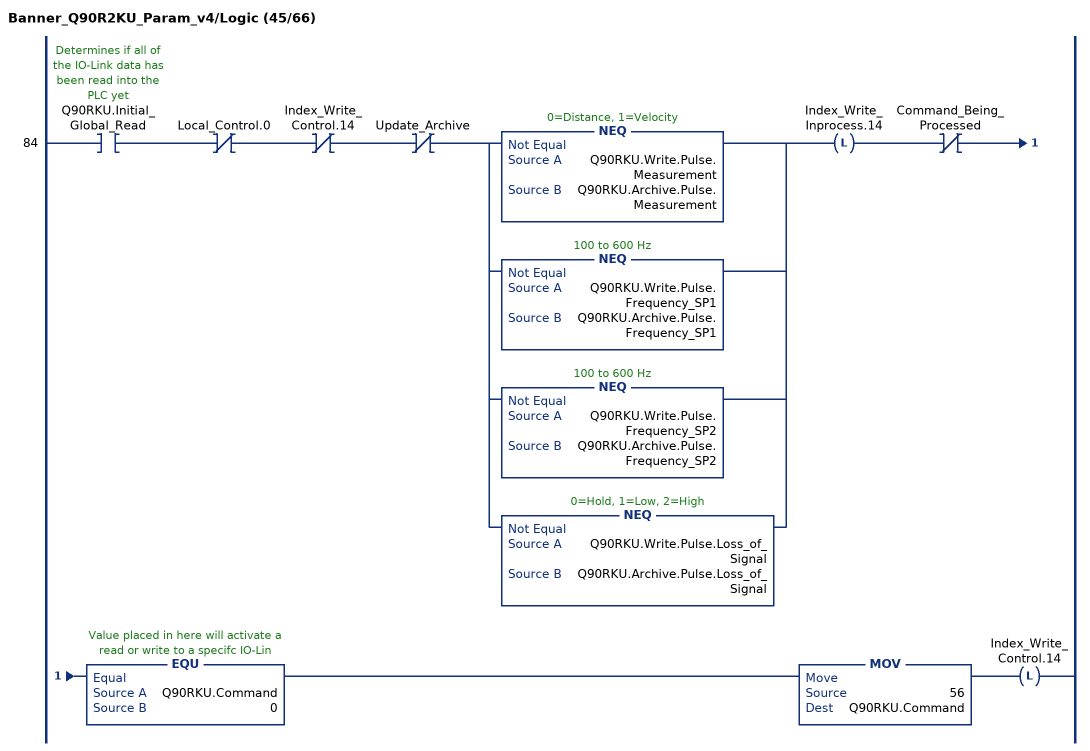
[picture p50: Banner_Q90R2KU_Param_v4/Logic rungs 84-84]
   84: XIC(Q90RKU.Initial_Global_Read)XIO(Local_Control.0)XIO(Index_Write_Control.14)XIO(Update_Archive)[NEQ(Q90RKU.Write.Pulse.Measurement,Q90RKU.Archive.Pulse.Measurement) ,NEQ(Q90RKU.Write.Pulse.Frequency_SP1,Q90RKU.Archive.Pulse.Frequency_SP1) ,NEQ(Q90RKU.Write.Pulse.Frequency_SP2,Q90RKU.Archive.Pulse.Frequency_SP2) ,NEQ(Q90RKU.Write.Pulse.Loss_of_Signal,Q90RKU.Archive.Pulse.Loss_of_Signal) ]OTL(Index_Write_Inprocess.14)XIO(Command_Being_Processed)EQU(Q90RKU.Command,0)MOV(56,Q90RKU.Command)OTL(Index_Write_Control.14);
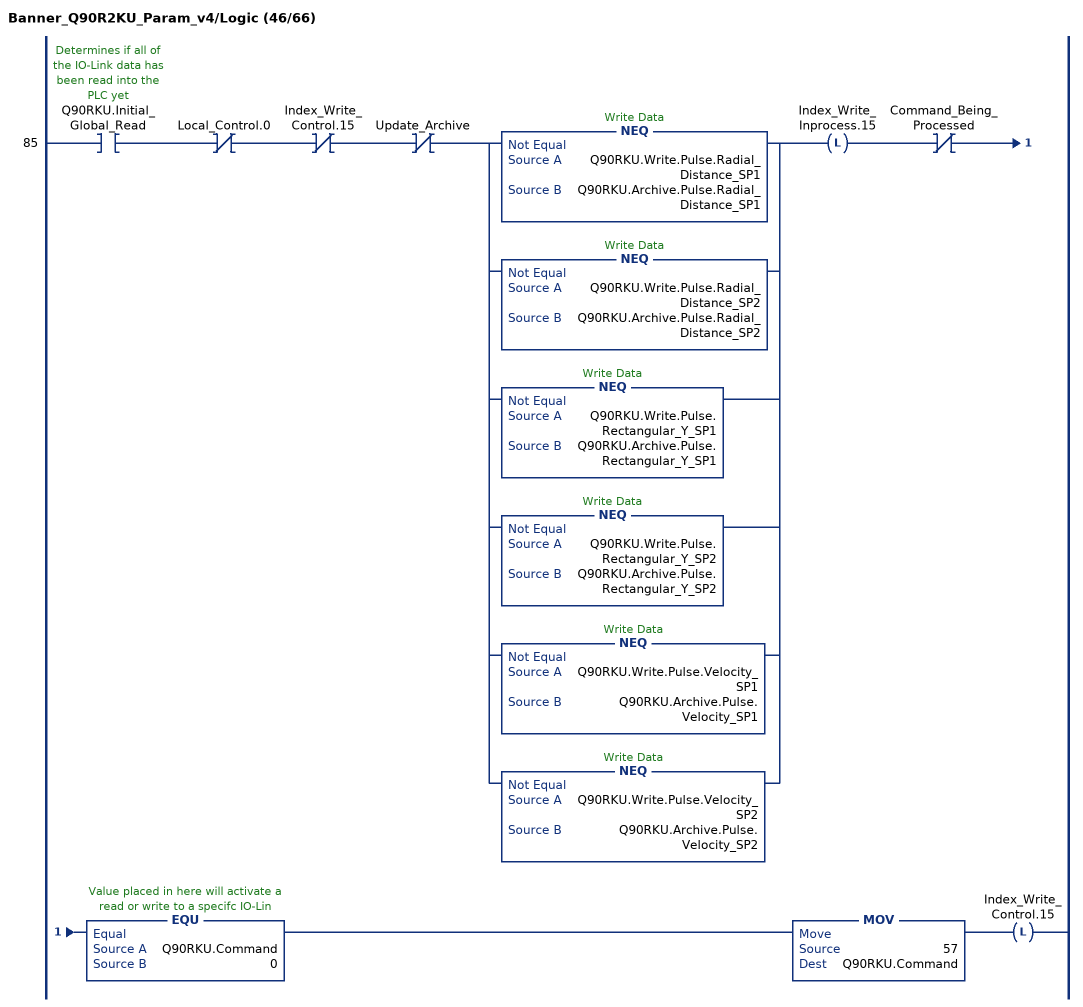
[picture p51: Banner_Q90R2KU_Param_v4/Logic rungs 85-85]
   85: XIC(Q90RKU.Initial_Global_Read)XIO(Local_Control.0)XIO(Index_Write_Control.15)XIO(Update_Archive)[NEQ(Q90RKU.Write.Pulse.Radial_Distance_SP1,Q90RKU.Archive.Pulse.Radial_Distance_SP1) ,NEQ(Q90RKU.Write.Pulse.Radial_Distance_SP2,Q90RKU.Archive.Pulse.Radial_Distance_SP2) ,NEQ(Q90RKU.Write.Pulse.Rectangular_Y_SP1,Q90RKU.Archive.Pulse.Rectangular_Y_SP1) ,NEQ(Q90RKU.Write.Pulse.Rectangular_Y_SP2,Q90RKU.Archive.Pulse.Rectangular_Y_SP2) ,NEQ(Q90RKU.Write.Pulse.Velocity_SP1,Q90RKU.Archive.Pulse.Velocity_SP1) ,NEQ(Q90RKU.Write.Pulse.Velocity_SP2,Q90RKU.Archive.Pulse.Velocity_SP2) ]OTL(Index_Write_Inprocess.15)XIO(Command_Being_Processed)EQU(Q90RKU.Command,0)MOV(57,Q90RKU.Command)OTL(Index_Write_Control.15);
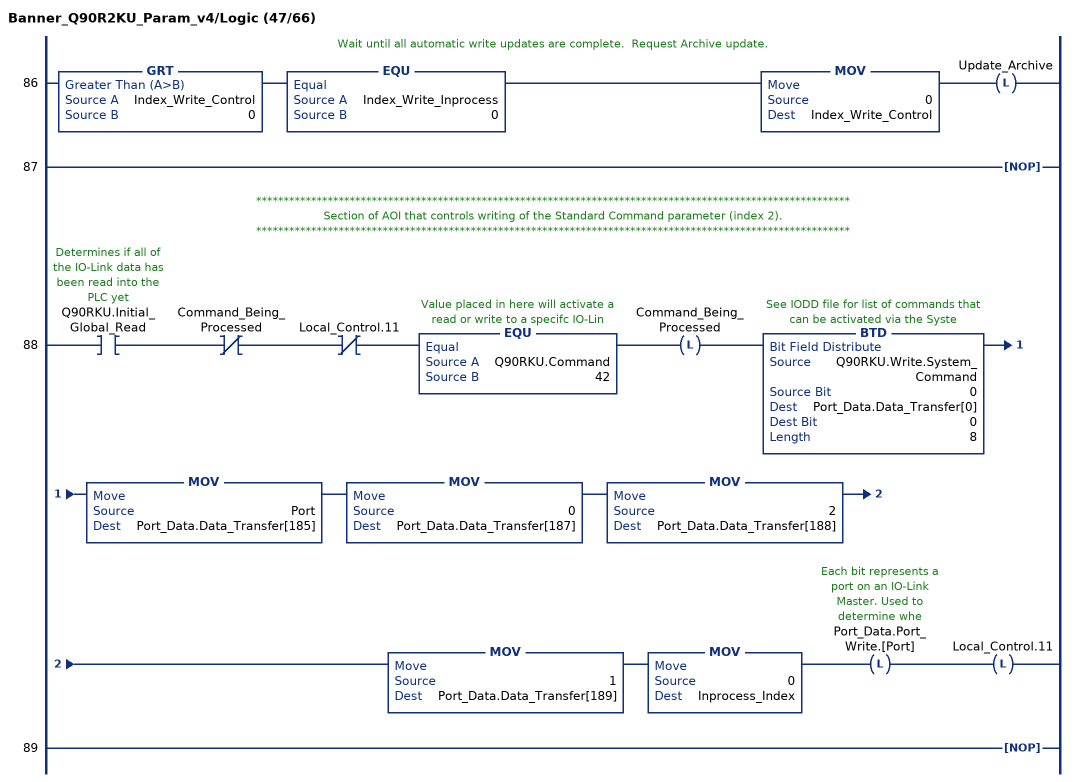
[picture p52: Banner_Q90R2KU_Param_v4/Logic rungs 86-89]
   // Wait until all automatic write updates are complete.  Request Archive update.
   86: GRT(Index_Write_Control,0)EQU(Index_Write_Inprocess,0)MOV(0,Index_Write_Control)OTL(Update_Archive);
   87: NOP();
   // ************************************************************************************************************
   // Section of AOI that controls writing of the Standard Command parameter (index 2).
   // ************************************************************************************************************
   88: XIC(Q90RKU.Initial_Global_Read)XIO(Command_Being_Processed)XIO(Local_Control.11)EQU(Q90RKU.Command,42)OTL(Command_Being_Processed)BTD(Q90RKU.Write.System_Command,0,Port_Data.Data_Transfer[0],0,8)MOV(Port,Port_Data.Data_Transfer[185])MOV(0,Port_Data.Data_Transfer[187])MOV(2,Port_Data.Data_Transfer[188])MOV(1,Port_Data.Data_Transfer[189])MOV(0,Inprocess_Index)OTL(Port_Data.Port_Write.[Port])OTL(Local_Control.11);
   89: NOP();
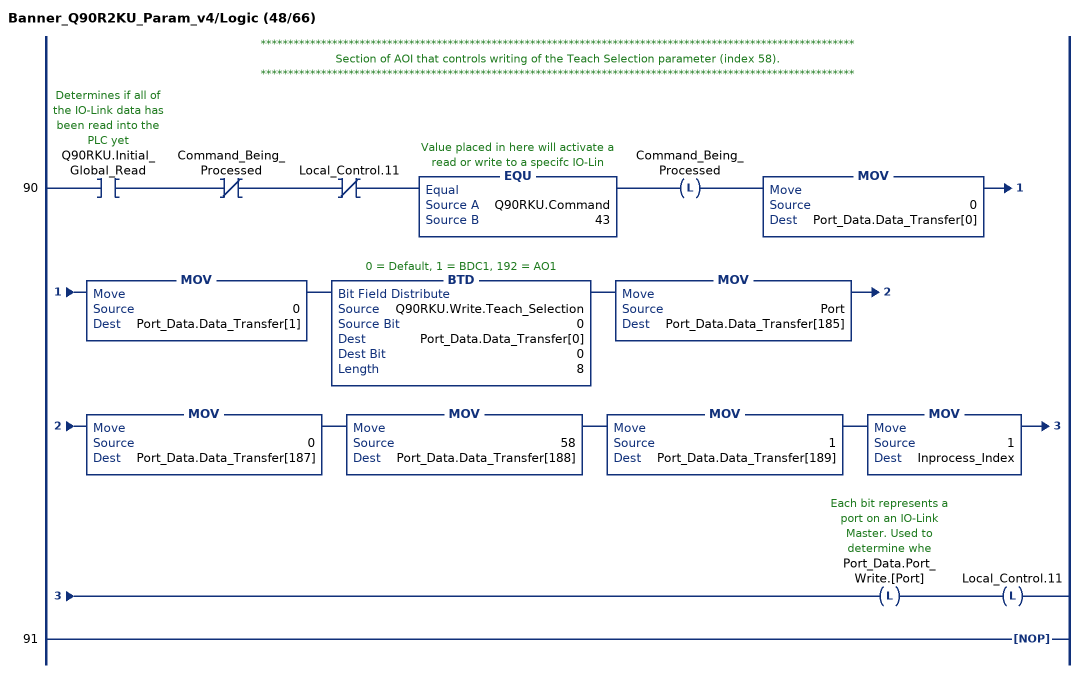
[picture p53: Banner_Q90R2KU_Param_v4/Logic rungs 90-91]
   // ************************************************************************************************************
   // Section of AOI that controls writing of the Teach Selection parameter (index 58).
   // ************************************************************************************************************
   90: XIC(Q90RKU.Initial_Global_Read)XIO(Command_Being_Processed)XIO(Local_Control.11)EQU(Q90RKU.Command,43)OTL(Command_Being_Processed)MOV(0,Port_Data.Data_Transfer[0])MOV(0,Port_Data.Data_Transfer[1])BTD(Q90RKU.Write.Teach_Selection,0,Port_Data.Data_Transfer[0],0,8)MOV(Port,Port_Data.Data_Transfer[185])MOV(0,Port_Data.Data_Transfer[187])MOV(58,Port_Data.Data_Transfer[188])MOV(1,Port_Data.Data_Transfer[189])MOV(1,Inprocess_Index)OTL(Port_Data.Port_Write.[Port])OTL(Local_Control.11);
   91: NOP();
